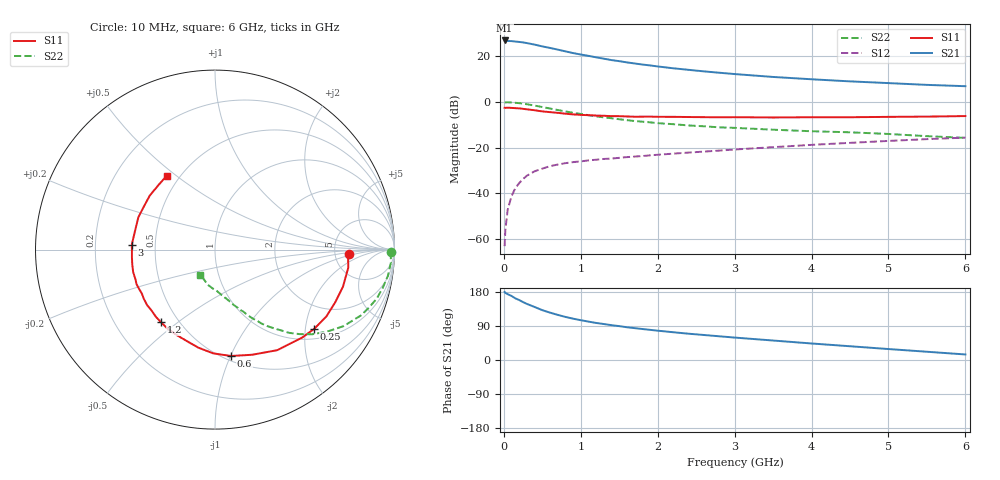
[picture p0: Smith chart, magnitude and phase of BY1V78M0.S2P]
! SIEMENS Small Signal Semiconductors
! BFY420
! Si NPN RF SIEGET Grounded Emitter Transistor in MICRO-X
! VCE = 1.75 V  IC = 8 mA
! Common Emitter S-Parameters:  October  1996
# GHz  S  MA  R  50
!  f  S11  S21  S12  S22
! GHz  MAG  ANG  MAG  ANG  MAG  ANG  MAG  ANG
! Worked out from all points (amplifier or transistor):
!   36 points, 10 MHz to 6 GHz, reference 50 ohm
!   highest |S21| = 26.9 dB at 10 MHz (marker M1)
!   |S21| within 3 dB of that: start of sweep to 560 MHz
!   unconditionally stable (mu >= 1): 2.66 GHz to end of sweep
!   at 250 MHz: K = 0.15, MSG = 29.9 dB, |S12| = -33.7 dB
!   at 1.4 GHz: K = 0.69, MSG = 21.5 dB, |S12| = -24.8 dB
!   at 6 GHz: K = 1.12, MAG = 9.1 dB, |S12| = -15.6 dB
!   S11 on the Smith chart (normalised r, x): 10 MHz: 6.84, -0.73; 250 MHz: 1.27, -2.24; 600 MHz: 0.54, -1.00; 1.2 GHz: 0.40, -0.44; 3 GHz: 0.37, +0.02; 6 GHz: 0.43, +0.46
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0.01  0.7474 -1.8  22.16 179.5  0.0007 106.2  0.9831 -0.8
0.02  0.7431 -3.6  22.02 177.1  0.0016 83.4  0.9797 -1.5
0.05  0.7494 -7.7  21.57 173.7  0.0044 83.0  0.9826 -4.2
0.1  0.7424 -16.1  21.47 169.0  0.0087 82.7  0.9744 -8.6
0.15  0.7315 -23.6  20.96 162.6  0.0131 77.9  0.9589 -12.8
0.2  0.7239 -30.9  20.58 158.2  0.0168 75.7  0.942 -16.8
0.25  0.7075 -38.6  20.06 152.7  0.0206 71.7  0.9162 -20.7
0.3  0.69 -45.3  19.41 148.0  0.0244 68.8  0.8919 -24.3
0.4  0.6588 -58.3  17.98 139.9  0.0304 62.8  0.8332 -30.8
0.5  0.6212 -70.6  16.43 131.5  0.0348 58.9  0.7739 -36.2
0.6  0.5993 -81.5  15.21 125.0  0.0394 55.3  0.7189 -41.0
0.8  0.5542 -99.6  12.8 113.7  0.0458 50.2  0.6212 -48.3
0.9  0.5344 -106.6  11.74 109.1  0.0483 48.4  0.5802 -50.8
1.1  0.5138 -120.9  10.2 101.3  0.0527 46.4  0.5143 -55.8
1.2  0.504 -126.7  9.48 97.8  0.0546 45.7  0.4854 -57.9
1.6  0.4819 -145.6  7.336 86.4  0.0621 43.9  0.3996 -64.1
2.2  0.4729 -164.7  5.462 73.3  0.074 42.3  0.3268 -71.2
3  0.4645 176.7  4.081 59.2  0.0912 40.7  0.2712 -78.8
3.5  0.4576 166.2  3.525 51.4  0.1026 38.8  0.2474 -83.5
4.5  0.4633 148.9  2.822 36.3  0.1274 33.1  0.2169 -93.4
5.5  0.4781 131.1  2.365 21.8  0.1537 25.7  0.1787 -109.6
6  0.4914 123.2  2.212 14.6  0.166 21.6  0.1637 -120.6
